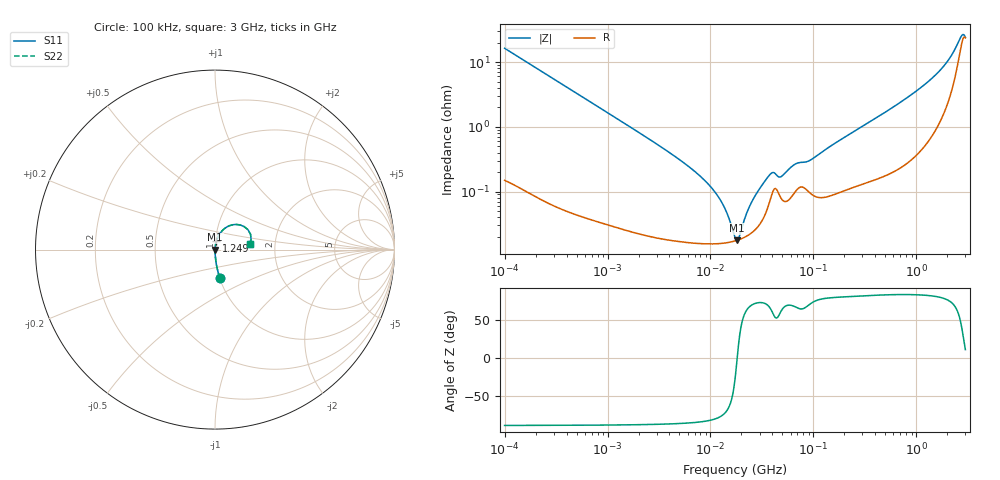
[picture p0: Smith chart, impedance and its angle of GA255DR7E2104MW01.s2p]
!Murata Part Number: GA255DR7E2104MW01
!These Parameters are Measured in Series Mode Connection
!Data Generated on Jun 19, 2026
!  o--ll--o
!Port1  Port2
!  o------o
!Operation Temp=25[degC], DC Bias Voltage=0[V]
!Freq. Start=100[kHz] Stop=3[GHz] 401[Steps]
# Hz S RI R 50
!Freq.(Hz) S11(Real) S11(Imag) S21(Real) S21(Imag) S12(Real) S12(Imag) S22(Real) S22(Imag)
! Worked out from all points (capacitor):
!   401 points, 100 kHz to 3 GHz, reference 50 ohm
!   read as one part in series: C = 97.1 nF near 105.3 kHz
!   lowest |Z| = 17.7 mohm at 18.24 MHz (marker M1)
!   series resonance near 18.19 MHz, so ESL is about 790 pH
!   S11 on the Smith chart (normalised r, x): 100 kHz: 1.00, -0.33; 1.249 GHz: 1.01, +0.09; 3 GHz: 1.47, +0.09
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100000  0.0275 -0.1589  0.9725 0.1589  0.9725 0.1589  0.0275 -0.1589
562235  0.00127 -0.0293  0.9987 0.0293  0.9987 0.0293  0.00127 -0.0293
3161081  0.000215 -0.00513  0.9998 0.00513  0.9998 0.00513  0.000215 -0.00513
6674626  0.000165 -0.00219  0.9998 0.00219  0.9998 0.00219  0.000165 -0.00219
1.034438e7  0.000156 -0.00111  0.9998 0.00111  0.9998 0.00111  0.000156 -0.00111
1.37349e7  0.00016 -0.000536  0.9998 0.000536  0.9998 0.000536  0.00016 -0.000536
1.77727e7  0.000174 -4.37e-05  0.9998 4.37e-05  0.9998 4.37e-05  0.000174 -4.37e-05
1.82367e7  0.000177 5.4e-06  0.9998 -5.4e-06  0.9998 -5.4e-06  0.000177 5.4e-06
1.920135e7  0.000182 0.000104  0.9998 -0.000104  0.9998 -0.000104  0.000182 0.000104
2.241242e7  0.000204 0.000408  0.9998 -0.000408  0.9998 -0.000408  0.000204 0.000408
2.549486e7  0.000235 0.000678  0.9998 -0.000678  0.9998 -0.000678  0.000235 0.000678
3.752708e7  0.000692 0.00166  0.9993 -0.00166  0.9993 -0.00166  0.000692 0.00166
4.054368e7  0.00101 0.00169  0.999 -0.00169  0.999 -0.00169  0.00101 0.00169
4.855934e7  0.000789 0.0015  0.9992 -0.0015  0.9992 -0.0015  0.000789 0.0015
6.615861e7  0.00098 0.00245  0.999 -0.00245  0.999 -0.00245  0.00098 0.00245
9.738194e7  0.0009 0.00305  0.9991 -0.00305  0.9991 -0.00305  0.0009 0.00305
5.475153e8  0.0022 0.0183  0.9978 -0.0183  0.9978 -0.0183  0.0022 0.0183
1.24901e9  0.00752 0.0462  0.9925 -0.0462  0.9925 -0.0462  0.00752 0.0462
1.838476e9  0.0222 0.0812  0.9778 -0.0812  0.9778 -0.0812  0.0222 0.0812
2.504792e9  0.1007 0.1387  0.8993 -0.1387  0.8993 -0.1387  0.1007 0.1387
2.776789e9  0.1831 0.1113  0.8169 -0.1113  0.8169 -0.1113  0.1831 0.1113
3e9  0.1925 0.031  0.8075 -0.031  0.8075 -0.031  0.1925 0.031
